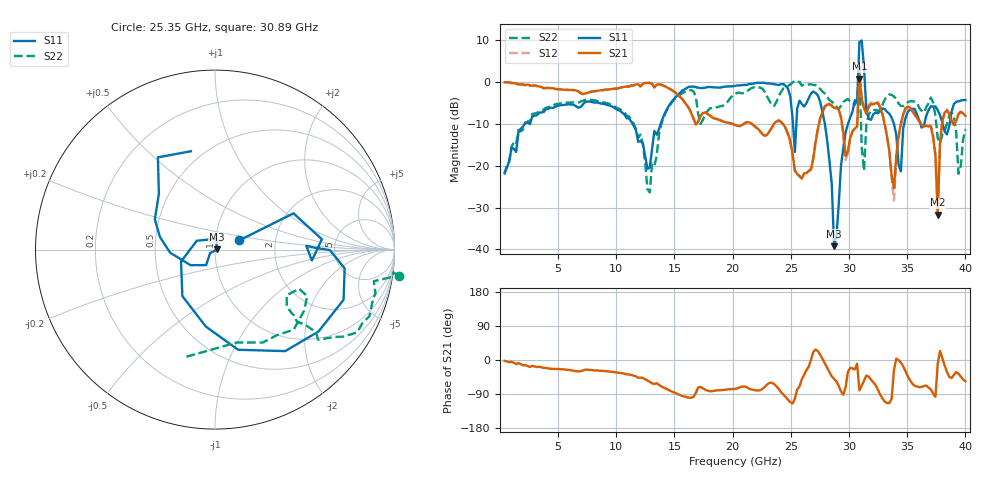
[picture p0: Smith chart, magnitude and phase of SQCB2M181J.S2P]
! Network Analyzer HP8722ES.07.66: Jul 25, 2000 Serial No. US39175408
! 27 Oct 2004  13:19:10
! Frequency  S11  S21  S12  S22
# HZ  S  DB R  50
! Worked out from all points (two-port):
!   201 points, 400 MHz to 40 GHz, reference 50 ohm
!   highest |S21| = 0.75 dB at 30.89 GHz (marker M1); lowest = -31.7 dB at 37.62 GHz (marker M2)
!   |S21| within 3 dB of the highest: start of sweep to 6.721 GHz; 8.058 GHz to 14.94 GHz (6.877 GHz wide, 59.8 % of centre)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
!   lowest |S11| = -39.2 dB at 28.71 GHz (marker M3), VSWR 1.02, Z = 51.1 + j0.129 ohm
!   |S11| at or under -10 dB: start of sweep to 2.118 GHz; 11.4 GHz to 13.81 GHz (2.415 GHz wide, 19.2 % of centre); 27.92 GHz to 29.91 GHz (1.986 GHz wide, 6.87 % of centre)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
!   |S22| runs from -26.4 to 2.6 dB; largest |S21 - S12| = 0.55
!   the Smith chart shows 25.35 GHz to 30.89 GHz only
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4e8  -21.63 -97.7  -0.07 -2.4  -0.04 -1.8  -22.16 -95.4
7.132e9  -5.37 -100.1  -2.87 -27.4  -2.96 -28.4  -4.49 -117.7
1.2874e10  -20.46 -17.7  -0.24 -57.4  -0.23 -58.4  -26.38 57.2
1.3666e10  -11.30 7.3  -0.56 -65.7  -0.54 -66.2  -12.47 28.4
2.02e10  -0.92 4.3  -10.28 -76.2  -10.31 -77.0  -2.86 -8.0
2.4556e10  -0.98 -24.7  -11.00 -97.9  -11.26 -99.1  -1.17 2.7
2.5348e10  -16.73 20.8  -21.13 -102.0  -21.36 -101.0  0.29 -8.1
2.6932e10  -2.28 -21.3  -18.35 21.5  -17.90 21.3  -0.75 -26.6
2.812e10  -13.95 -160.6  -5.43 -21.0  -5.20 -24.5  -3.52 -39.7
2.8714e10  -39.22 6.6  -6.19 -49.5  -6.12 -52.4  -5.17 -39.6
3.0694e10  -4.97 103.8  -10.69 -10.0  -10.50 -8.8  -4.18 -105.0
3.0892e10  9.50 80.5  0.75 -80.0  4.22 -74.2  2.57 76.4
3.109e10  9.90 -79.4  -3.94 -67.8  -3.78 -66.7  -15.59 -156.3
3.1288e10  3.37 -109.6  -6.33 -54.2  -5.93 -52.5  -21.22 -47.2
3.1486e10  -6.58 -107.7  -7.58 -41.2  -6.96 -41.5  -10.36 12.7
3.3466e10  -7.61 174.2  -16.57 -113.6  -16.65 -121.1  -2.98 -25.6
3.3862e10  -10.04 153.5  -25.34 -26.5  -28.26 -21.0  -3.47 -52.3
3.4456e10  -21.36 -98.8  -9.94 -6.9  -10.48 -4.3  -5.74 -86.2
3.703e10  -5.80 -171.0  -10.64 -77.6  -10.42 -75.6  -3.71 124.7
3.7624e10  -6.74 170.0  -31.67 -9.1  -30.36 -5.2  -13.46 95.5
3.8218e10  -11.84 176.8  -7.33 -14.6  -7.12 -15.5  -11.69 143.4
4e10  -4.33 -172.8  -8.10 -56.0  -8.14 -56.4  -11.37 165.0
